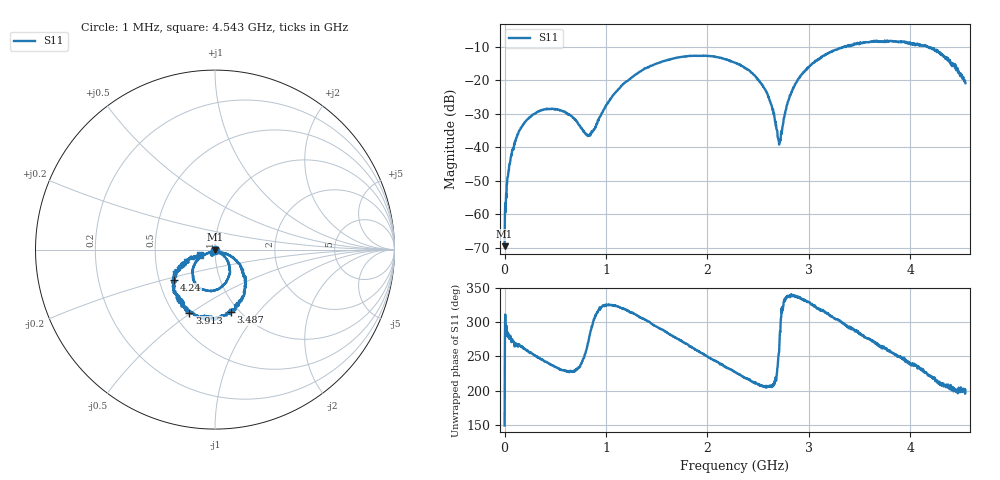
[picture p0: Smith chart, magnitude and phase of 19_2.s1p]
# HZ S RI R 50
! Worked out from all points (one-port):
!   1515 points, 1 MHz to 4.543 GHz, reference 50 ohm
!   lowest |S11| = -69.5 dB at 1 MHz (marker M1), VSWR 1.00, Z = 50 + j0.0173 ohm
!   |S11| at or under -10 dB: start of sweep to 3.342 GHz; 3.357185 GHz to 3.361632 GHz (4.448 MHz wide, 0.132 % of centre); 4.173 GHz to end of sweep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
!   S11 on the Smith chart (normalised r, x): 1 MHz: 1.00, +0.00; 3.487 GHz: 0.91, -0.73; 3.913 GHz: 0.60, -0.49; 4.24 GHz: 0.60, -0.22; 4.543 GHz: 0.84, -0.05
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1000000  -0.000289 0.000173
2.5e7  0.000477 -0.00279
4.9e7  0.000979 -0.00558
8.5e7  0.000197 -0.00974
1.48e8  -0.00103 -0.018
3.43e8  -0.0133 -0.0323
5.71e8  -0.0225 -0.0267
8.35e8  0.00231 -0.0151
1.138e9  0.0611 -0.048
1.381e9  0.0839 -0.125
1.705e9  0.0224 -0.2177
2.038e9  -0.0923 -0.2095
2.272e9  -0.1247 -0.1347
2.428e9  -0.1101 -0.0748
2.563e9  -0.0675 -0.0331
2.638e9  -0.035 -0.0164
2.692e9  -0.00834 -0.0117
2.71e9  -3.9e-05 -0.0118
2.782e9  0.0394 -0.016
2.842e9  0.0697 -0.0267
3.046e9  0.149 -0.1061
3.409e9  0.125 -0.3037
3.487e9  0.0895 -0.3493
3.913e9  -0.1438 -0.3531
3.976e9  -0.1707 -0.3146
4.24e9  -0.229 -0.1686
4.441e9  -0.1446 -0.051
4.543e9  -0.085 -0.0323
